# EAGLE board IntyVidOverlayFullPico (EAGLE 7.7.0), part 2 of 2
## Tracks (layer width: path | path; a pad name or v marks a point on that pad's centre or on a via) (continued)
RDBUS  (via drill 0.25) (continued)
  Bottom 0.254: v44.61,60.01 45.24,60.01 47.31,62.07 47.31,77.15 47.94,77.79 47.94,79.06 46.99,80.01 46.99,100.65 49.21,102.87 49.21,120.97 49.53,121.28 49.53,125.09 49.05,125.57 49.05,128.59 52.07,131.6 v52.07,131.76 | v133.67,131.76 139.22,131.76 140.02,132.56 IC7.11
RDENBL
  Top 0.254: IC12.9 176.53,134.62 173.67,137.48 152.4,137.48 | 152.4,137.48 146.21,137.48 145.1,136.37 IC7.9 | TP2.TP 152.4,137.48
  Bottom 0.254: IC12.9 176.53,132.08 175.26,130.81 175.26,116.2 173.99,114.94 IC19.7 173.99,106.2 163.83,96.04 163.83,87 164.15,86.68 164.15,85.41 162.56,83.82 IC15.5 | IC18.3 IC18.12 137.48,123.19 | IC7.1 132.4,125.09 133.35,124.14 136.53,124.14 137.48,123.19 | IC7.9 145.1,132.72 141.29,128.91 139.38,128.91 138.75,128.27 138.75,124.46 137.48,123.19
READP  (via drill 0.25)
  Top 0.254: IC22.3 34.29,69.69 33.34,70.64 28.89,70.64 v27.94,71.6 | v26.67,84.77 24.13,84.77 v22.7,86.2 | v23.34,114.78 26.99,114.78 30.48,118.27 34.29,118.27 | 34.29,118.27 IC31.2 | IC31.4 39.37,116.84 37.94,118.27 34.29,118.27
  Bottom 0.254: v27.94,71.6 27.94,72.39 26.67,73.66 v26.67,84.77 | v22.7,86.2 20.64,88.27 20.64,112.08 v23.34,114.78
READPD  (via drill 0.25)
  Top 0.254: v40.64,117.47 v40.64,120.97 | v40.64,137.48 40.8,137.64 43.02,137.64 43.5,137.16 45.24,137.16 45.72,137.64 49.37,137.64 50.32,138.59 52.55,138.59 53.18,139.22 57.47,139.22 58.42,138.27 IC8.19
  Bottom 0.254: IC31.3 36.83,116.68 37.78,117.63 40.48,117.63 v40.64,117.47 | v40.64,120.97 v40.64,137.48
READPS  (via drill 0.25)
  Top 0.254: v91.6,139.7 93.5,137.79 95.89,137.79 96.84,136.84 96.84,135.57 96.2,134.94 93.19,134.94 91.92,133.67 IC20.19
  Bottom 0.254: IC31.6 44.45,119.22 45.72,120.49 45.72,143.99 48.26,146.53 87.95,146.53 91.6,142.88 v91.6,139.7
RF  (via drill 0.25)
  Top 0.254: IC29.13 157.48,41.27 TP6.TP v160.02,46.35
  Bottom 0.254: IC15.9 165.1,87.63 166.37,86.36 166.37,76.83 163.83,74.3 163.83,69.22 166.37,66.67 166.37,61.91 160.02,55.56 v160.02,46.35
RF'  (via drill 0.25)
  Top 0.254: v131.44,27.46 151.61,27.46 154.94,30.8 IC29.7
  Bottom 0.254: JP2.10 108.27,33.97 113.67,33.97 117.47,30.16 128.75,30.16 v131.44,27.46
RUN
  Bottom 0.254: JP2.11 114.46,40.8 PB1.1
SELA  (via drill 0.25)
  Top 0.254: v50.48,131.76 50.48,131.13 53.5,128.11 53.5,125.25 51.91,123.67 51.91,120.33 53.02,119.22 54.13,119.22 54.53,119.62 70.17,119.62 70.64,120.09 70.64,123.03 71.75,124.14 79.85,124.14 80.8,123.19 80.8,120.65 81.76,119.7 87.79,119.7 88.42,119.06 88.42,118.11 89.38,117.16 115.57,117.16 128.91,130.49 134.3,130.49 134.94,131.13 IC7.13 | v44.77,71.75 46.04,73.03 46.04,77.15 45.4,77.79 42.86,77.79 41.91,76.83 IC22.9 | v48.42,28.1 54.13,28.1 55.09,29.05 56.67,29.05 58.42,30.8 IC28.17 | IC21.3 36.83,126.36 37.78,125.41 42.23,125.41 43.18,124.46 43.18,121.6 45.4,119.38 v46.67,119.38
  Bottom 0.254: IC22.9 41.91,77.79 43.18,79.06 43.18,98.42 48.26,103.5 48.26,117.79 v46.67,119.38 46.67,119.86 48.58,121.76 48.58,124.46 48.1,124.94 48.1,129.38 v50.48,131.76 | v44.77,71.75 43.18,70.17 43.18,59.21 46.35,56.04 46.35,52.7 45.09,51.44 45.09,31.43 v48.42,28.1
SELA'
  Top 0.254: JP2.12 109.22,33.02 98.27,33.02 94.77,29.53 76.52,29.53 72.87,25.88 57.63,25.88 55.88,24.13 IC28.3
SELB  (via drill 0.25)
  Top 0.254: IC16.3 34.29,81.28 33.02,80.01 29.37,80.01 v29.21,79.85 | v27.94,65.72 28.26,65.41 30.32,65.41 31.75,63.98 IC23.13 | v48.1,26.19 48.42,26.19 49.21,26.99 55.88,26.99 56.83,27.94 61.75,27.94 63.5,29.69 IC28.15 | v35.56,91.6 35.08,92.08 30.96,92.08 29.21,93.82 IC24.1
  Bottom 0.254: IC23.13 31.75,61.28 35.56,57.47 35.56,53.02 36.2,52.39 39.37,52.39 | 39.37,52.39 IC23.5 | v29.21,79.85 27.62,78.34 27.62,74.3 29.21,72.71 29.21,70.8 27.62,69.22 27.62,66.04 v27.94,65.72 | 39.37,52.39 42.86,48.9 42.86,31.43 v48.1,26.19 | IC16.3 34.29,85.72 35.56,87 v35.56,91.6 35.88,91.92 36.51,91.92 38.1,93.5 38.1,110.17 41.91,113.98 IC31.5
SELB'  (via drill 0.25)
  Top 0.254: v118.11,33.5 115.09,30.48 97.63,30.48 94.3,27.15 84.93,27.15 81.92,24.13 78.26,24.13 75.88,21.75 61.59,21.75 60.96,22.38 IC28.5
  Bottom 0.254: JP2.19 127.48,33.5 v118.11,33.5
SELECT
  Top 0.254: IC20.15 90.33,123.51 87,126.84 87,137 86.84,137.16 86.84,138.43 89.38,140.97 X1.13
TSCLK
  Top 0.254: IC19.10 173.99,122.56 172.72,123.83 172.72,127 171.45,128.27 159.07,128.27 158.12,129.22 152.08,129.22 151.61,129.7 139.54,129.7 137.48,127.64 IC7.3
VBUS  (via drill 0.61)
  Top 1.27: Q1.G 116.84,47.15 114.14,44.45 v88.11,44.45
  Bottom 1.27: v88.11,44.45 83.82,40.16 JP2.1
VCC  (via drill 0.61)
  Top 0.254: IC1.26 94.14,60.01 89.06,60.01 88.74,60.33 86.68,60.33 86.04,59.69 86.04,56.2
  Top 1.27: IC23.14 C23.1 | IC22.14 v25.08,75.56 C22.1 | v127.32,133.35 132.4,133.35 IC7.14 132.4,136.68 C7.1 132.56,137.79 v136.68,141.92 | IC14.13 IC14.12 IC14.11 IC14.10 | IC13.11 IC13.10 | IC13.15 IC13.16 | IC12.11 171.45,131.44 170.18,130.18 166.37,130.18 | 166.37,130.18 IC12.13 | 166.37,130.18 v161.29,130.18 | IC14.15 IC14.16 | v79.22,44.45 76.99,44.45 73.66,41.12 v51.44,41.12 47.94,41.12 46.67,42.39 v38.89,42.39 | IC15.7 167.64,77.79 165.42,75.56 v160.66,75.56 150.81,75.56 v149.54,76.83 137.16,76.83 v135.89,75.56 C13.1 | v49.85,68.58 IC5.20 53.02,68.9 C5.1 | 105.41,89.85 IC11.14 C11.1 | 105.41,89.85 v125.73,89.85 | 87.15,89.85 85.41,89.85 C10.1 IC10.14 | 87.15,89.85 105.41,89.85 | C24.1 23.18,102.87 v24.77,102.87 IC24.14 | IC2.14 148.27,71.75 C2.1 | IC12.16 IC12.15 | IC12.4 IC12.5 | R14.P$2 87.15,89.85 | IC1.32 86.04,56.2 C1.1 v82.07,56.2 | IC31.14 26.83,123.03 v26.67,122.87 | IC21.14 31.75,134.3 33.5,132.56 48.26,132.56 50.16,134.46 52.55,134.46 53.34,135.25 C8.1 | C25.1 55.4,123.19 IC25.20 | IC24.4 IC24.3
  Bottom 1.27: 51.44,57.15 51.44,52.7 50.16,51.44 50.16,46.35 51.44,45.09 v51.44,41.12 | 51.44,57.15 51.44,60.96 49.85,62.55 v49.85,68.58 49.85,75.56 51.12,76.83 51.12,82.55 51.44,82.87 51.44,87.95 | 51.44,87.95 51.44,97.79 | 51.44,97.79 51.44,98.11 52.39,99.06 | 52.39,99.06 52.39,115.89 51.91,116.36 51.91,121.44 C25.1 53.66,130.97 55.72,133.03 IC8.20 C8.1 | IC4.20 51.44,87.95 | IC3.20 51.44,57.15 | C23.1 25.88,63.02 25.88,72.23 25.08,73.03 v25.08,75.56 25.08,79.38 24.77,79.69 24.77,90.49 | 24.77,90.49 v24.77,102.87 24.77,108.58 26.35,110.17 FB1.P$2 26.35,121.6 | 26.35,121.6 26.35,122.56 v26.67,122.87 26.67,132.72 C21.1 IC21.14 | 156.21,121.28 156.21,100.49 149.86,94.14 149.86,85.09 148.59,83.82 148.59,77.79 v149.54,76.83 149.22,76.52 149.22,72.71 C2.1 | 156.21,121.28 156.21,121.6 | 156.21,121.6 156.21,129.06 158.75,131.6 IC12.16 C12.1 156.37,138.59 151.45,143.51 138.27,143.51 v136.68,141.92 | IC12.15 v161.29,130.18 IC12.2 | IC19.16 156.21,121.28 | 127.32,137.48 v127.32,133.35 127.32,123.03 126.21,121.92 126.21,92.55 C14.1 v125.73,89.85 IC14.16 | 127.32,137.48 127.32,143.99 126.21,145.1 IC9.15 IC9.16 125.09,148.11 C9.1 | IC14.10 140.97,88.58 142.88,90.49 142.88,99.85 147.64,104.62 IC18.7 | IC13.11 138.43,73.03 v135.89,75.56 133.35,78.11 IC14.4 IC14.13 133.35,88.27 137.64,92.55 137.64,104.93 140.02,107.31 C18.1 IC18.4 | IC15.10 162.56,86.04 160.02,83.5 IC15.4 C15.1 160.02,76.2 v160.66,75.56 | 135.57,55.88 143.03,48.42 R12.P$1 | 135.57,55.88 133.35,58.1 | 133.35,58.1 IC13.4 | IC6.20 52.39,99.06 | IC14.15 IC14.2 C13.1 IC13.15 IC13.2 128.27,63.18 133.35,58.1 | IC17.20 83.82,76.83 83.03,77.63 83.03,82.39 85.09,84.45 IC10.14
  Bottom 1.27: IC24.4 36.83,96.52 34.13,99.22 31.27,99.22 29.21,101.28 IC24.14 | IC17.20 83.82,73.03 82.07,71.28 v82.07,56.2 82.07,47.31 v79.22,44.45 | C17.1 81.76,73.66 IC17.20 | C6.1 51.44,97.79 | C4.1 51.44,87.95 | C3.1 51.44,57.15 | IC12.4 IC12.13 | 24.77,90.49 25.08,90.17 C16.1 28.89,90.17 IC16.14 | C19.1 156.21,121.6 | Q1.D 131.29,49.69 132.4,50.8 132.4,52.7 135.57,55.88 | C31.1 26.35,121.6 | 127.32,137.48 IC9.12 IC9.5 115.57,137.48 114.3,136.21 103.19,136.21 | 103.19,136.21 IC30.20 98.74,136.21 97,137.95 93.03,137.95 IC20.20 | v38.89,42.39 38.1,42.39 27.15,53.34 27.15,56.99 28.57,58.42 28.57,61.28 29.21,61.91 IC23.14 | 103.19,136.21 102.71,136.53 C30.1 103.03,138.43
VDD
  Top 1.27: JP4.43 10.16,102.87 10.16,111.28 | 10.16,111.28 10.16,113.98 8.73,115.41 8.73,117.32 5.71,120.33 R1.P$1 | JP6.22 185.26,101.6 178.59,108.27 178.59,115.41 176.85,117.16 131.13,117.16 127.95,113.98 120.33,113.98 117.63,111.28 10.16,111.28
  Bottom 1.27: R1.P$1 6.99,124.46 6.99,142.88 PWRSUPP.6
VDD2
  Bottom 1.27: FB1.P$1 14.92,116.52 PWRSUPP.3
VENABL  (via drill 0.25)
  Top 0.254: IC15.12 157.48,90.17 156.53,91.12 150.65,91.12 150.34,90.81 TP3.TP 135.1,90.81 v133.99,91.92
  Bottom 0.254: v133.99,91.92 134.3,92.23 134.3,104.78 136.21,106.68 136.21,116.84 132.4,120.65 IC18.14
VON  (via drill 0.25)
  Top 0.254: IC2.4 160.02,63.18 158.59,61.75 151.61,61.75 150.18,63.18 v150.18,65.41
  Bottom 0.254: IC15.1 152.4,75.56 150.81,73.98 150.81,71.75 150.18,71.12 v150.18,65.41
VSYS  (via drill 0.61)
  Top 1.27: Q1.S v121.92,52.23 | v112.08,42.39 v91.28,42.39
  Bottom 1.27: v121.92,52.23 v112.08,42.39 | v91.28,42.39 86.36,37.47 JP2.2
WB  (via drill 0.25)
  Top 0.254: IC22.10 39.37,73.98 37.31,71.91 36.83,71.91 | 36.83,71.91 v30.48,71.91 29.37,73.03 27.62,73.03 24.13,69.53 24.13,59.69 v25.56,58.26 | IC22.4 36.83,71.91 | v49.21,35.4 40.96,35.4 v40.64,35.08 40.64,26.51 48.58,18.57 48.58,13.34 50.8,11.11 IC26.1 | v52.7,33.34 52.86,33.5 59.69,33.5 60.96,32.23 IC28.16
  Bottom 0.254: v30.48,71.91 30.48,92.08 29.84,92.71 28.57,92.71 26.35,94.93 26.35,107 28.26,108.9 28.26,124.14 30.8,126.68 31.43,126.68 31.75,127 IC21.1 | v40.64,35.08 40.64,37.62 25.4,52.86 25.4,58.1 v25.56,58.26 | v49.21,35.4 50.64,35.4 v52.7,33.34
WB0  (via drill 0.25)
  Top 0.254: IC23.3 34.29,53.66 35.24,52.7 44.77,52.7 47.31,55.24 47.31,59.37 53.66,65.72 56.2,65.72 57.15,66.67 57.15,70.17 57.78,70.8 77.15,70.8 77.95,70.01 v77.95,69.69
  Bottom 0.254: v77.95,69.69 77.95,60.17 76.2,58.42 IC3.11
WB1  (via drill 0.25)
  Top 0.254: IC16.5 39.37,83.66 40.96,85.25 46.2,85.25 48.58,82.87 53.98,82.87 54.61,82.23 54.61,77.15 60.01,71.75 73.34,71.75 v73.66,72.07
  Bottom 0.254: IC23.6 41.91,56.2 40.64,57.47 40.64,78.9 39.37,80.17 IC16.5 | IC4.11 76.2,86.68 74.93,85.41 74.93,73.34 v73.66,72.07
WB'  (via drill 0.25)
  Top 0.254: IC28.4 58.42,22.38 60.01,20.8 76.83,20.8 79.06,23.02 82.39,23.02 85.41,26.04 95.89,26.04 99.38,29.53 116.84,29.53 v119.22,31.91
  Bottom 0.254: v119.22,31.91 128.43,31.91 JP2.20
WF  (via drill 0.25)
  Top 0.254: 46.67,29.37 46.67,23.81 50.64,19.84 77.79,19.84 79.85,21.91 82.87,21.91 85.88,24.92 97.31,24.92 100.97,28.57 121.76,28.57 124.3,26.04 160.02,26.04 v167.8,33.81 | v172.72,50.8 164.94,58.58 v159.86,58.58 | TP11.TP 46.67,29.37 | IC28.18 53.66,29.05 49.69,29.05 49.37,29.37 46.67,29.37
  Bottom 0.254: v167.8,33.81 172.72,38.73 v172.72,50.8 | v159.86,58.58 158.75,59.69 158.75,66.36 154.94,70.17 IC2.13
WF'
  Top 0.254: JP2.7 94.14,30.64 76.04,30.64 72.23,26.83 57.15,26.83 56.2,25.88 54.77,25.88 53.34,24.45 IC28.2
WRBUS
  Top 0.254: IC23.2 31.75,56.2 32.7,57.15 36.83,57.15 | 36.83,57.15 IC23.4 | 36.83,57.15 44.77,57.15 46.04,58.42 46.04,64.45 45.09,65.41 43.18,65.41 41.91,66.67 IC22.6
WRITP  (via drill 0.25)
  Top 0.254: v44.61,92.87 36.35,92.87 36.2,93.03 32.54,93.03 31.75,93.82 IC24.2
  Bottom 0.254: IC22.8 44.45,79.06 46.04,80.64 46.04,91.44 v44.61,92.87
WRITPC  (via drill 0.25)
  Top 0.254: IC24.13 31.75,101.76 32.86,100.65 45.4,100.65 48.9,104.14 69.85,104.14 70.64,103.35 80.33,103.35 v80.64,103.66
  Bottom 0.254: v80.64,103.66 84.14,107.16 104.78,107.16 110.17,112.55 110.17,114.14 109.38,114.94 105.57,114.94 103.98,113.35 IC30.11
WRITPD  (via drill 0.25)
  Top 0.254: v44.13,138.59 45.72,140.18 45.72,143.99 47.62,145.89 52.07,145.89 v52.86,145.1
  Bottom 0.254: IC24.12 34.29,108.27 30.16,112.39 30.16,117.16 32.7,119.7 41.59,119.7 43.18,121.28 43.18,137.64 v44.13,138.59 | IC25.11 79.53,122.87 78.42,123.98 78.42,126.68 80.01,128.27 80.01,134.62 80.49,135.1 80.49,138.59 79.85,139.22 79.85,141.6 78.58,142.88 78.58,144.62 77.79,145.41 53.18,145.41 v52.86,145.1

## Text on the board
tPlace: 4.7VDC MIN / 9VDC MAX | !HON | CLK4 | !HOFF | NTSC | RDENBL | (5VDC 2A OUT) | PIXCLK | VID / OUT | 44 | 43 | LV0 | LV3 | LV1 | LV2 | LV4 | LV7 | LV5 | LV6 | VENABL | CARTRIDGE PORT | To IntyQuadClockTap / (places PLL-locked / MCLKx4 ~ 14.31818 MHz / on pin 16 instead of GND) | DISPLAY | GND | L4 | L1 | L7 | LCH | DSP | L0 | L3 | L5 | L2 | L6 | !SR1 | DIGITAL / VIDEO OUT | Power / LED | + | - | 2 | 1 | RF | PI PICO / RESET | 40 | 21 | LOW-VOLT / VERSION!!! | WF | Raspberry Pi Pico | LOW-VOLT / VERSION!!! | !SR1 | 1 | 20 | CBLNK | LOW-VOLT / VERSION!!! | MUST use LVC low-volt versions or / you will FRY your Raspberry Pi Pico / and/or the four chips!!! | LOW-VOLT / VERSION!!! | Inty Video Overlay "Pico" | v1.2
bPlace: MCLK4 | 16 | 1 JAN 2022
